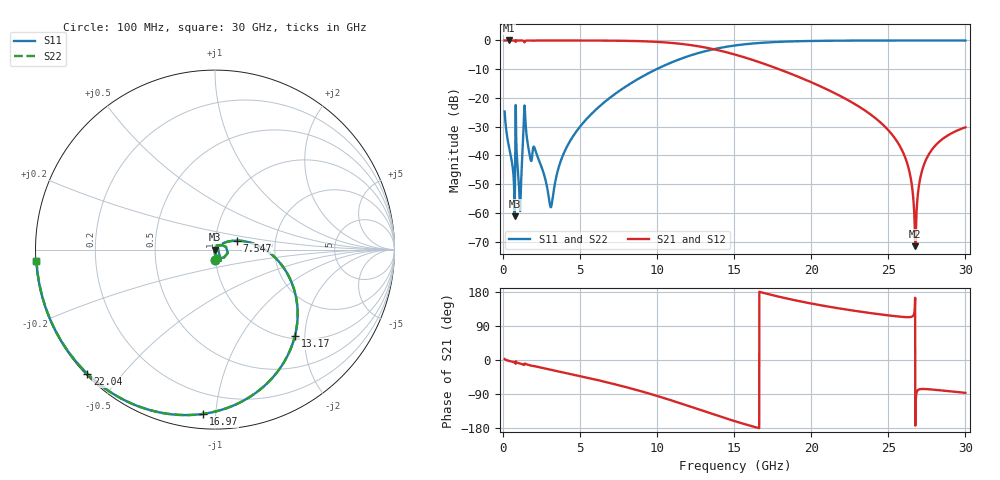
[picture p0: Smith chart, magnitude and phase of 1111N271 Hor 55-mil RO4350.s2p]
# GHz S MA R 50
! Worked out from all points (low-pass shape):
!   3201 points, 100 MHz to 30 GHz, reference 50 ohm
!   highest |S21| = 0.00 dB at 408.3 MHz (marker M1); lowest = -71.5 dB at 26.75 GHz (marker M2)
!   |S21| within 3 dB of the highest: start of sweep to 13.63 GHz
!   lowest |S11| = -61.2 dB at 754.1 MHz (marker M3), VSWR 1.00, Z = 50.1 + j0.00871 ohm
!   |S11| at or under -10 dB: start of sweep to 9.954 GHz
!   |S22| runs from -61.2 to 0.0 dB; largest |S21 - S12| = 0
!   S11 on the Smith chart (normalised r, x): 100 MHz: 1.00, -0.12; 7.547 GHz: 1.27, +0.13; 13.17 GHz: 1.06, -1.78; 16.97 GHz: 0.08, -0.93; 22.04 GHz: 0.00, -0.41; 30 GHz: 0.00, -0.03
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0.1  0.05823 -87.3  0.9981 2.5  0.9981 2.5  0.05823 -87.3
0.4083438  0.01304 -91.0  0.9995 -2.7  0.9995 -2.7  0.01304 -91.0
0.7540625  0.000874 5.7  0.9991 -6.3  0.9991 -6.3  0.000874 5.7
1.109125  0.00108 -8.7  0.9988 -9.3  0.9988 -9.3  0.00108 -8.7
1.454844  0.03839 -74.7  0.9827 -10.1  0.9827 -10.1  0.03839 -74.7
1.735156  0.009948 -86.5  0.9968 -13.9  0.9968 -13.9  0.009948 -86.5
2.11825  0.0118 -88.0  0.9959 -17.0  0.9959 -17.0  0.0118 -88.0
3.108687  0.001264 -20.0  0.9984 -25.7  0.9984 -25.7  0.001264 -20.0
3.846844  0.009507 50.4  0.9983 -32.1  0.9983 -32.1  0.009507 50.4
5.089563  0.03414 44.5  0.9975 -43.2  0.9975 -43.2  0.03414 44.5
7.546969  0.1329 22.1  0.9884 -67.1  0.9884 -67.1  0.1329 22.1
10.06978  0.3272 -6.2  0.9411 -95.7  0.9411 -95.7  0.3272 -6.2
13.17191  0.6558 -47.3  0.7493 -136.9  0.7493 -136.9  0.6558 -47.3
15.05  0.818 -71.9  0.5683 -161.6  0.5683 -161.6  0.818 -71.9
16.97481  0.9172 -94.0  0.3895 176.3  0.3895 176.3  0.9172 -94.0
20.03956  0.9797 -121.6  0.1856 148.7  0.1856 148.7  0.9797 -121.6
22.03912  0.992 -135.7  0.1029 134.7  0.1029 134.7  0.992 -135.7
25.01978  0.997 -153.2  0.02715 117.6  0.02715 117.6  0.997 -153.2
26.20644  0.9974 -159.3  0.007557 113.0  0.007557 113.0  0.9974 -159.3
26.74837  0.9974 -161.9  0.0002653 -173.4  0.0002653 -173.4  0.9974 -161.9
27.608  0.9973 -166.0  0.01027 -77.1  0.01027 -77.1  0.9973 -166.0
30  0.9968 -176.5  0.0309 -86.7  0.0309 -86.7  0.9968 -176.5
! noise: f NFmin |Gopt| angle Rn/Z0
0.1  0.0006561  0.731  1.002  0.0004861
3.417  0.009199  0.4597  28.07  0.002716
6.743  0.01514  0.4075  51.35  0.003502
10.06  0.02326  0.4503  69.75  0.005088
13.39  0.03637  0.5543  86.66  0.008291
16.7  0.06215  0.6991  105.3  0.01566
20.03  0.1256  0.8391  125.5  0.03567
23.35  0.3497  0.939  144.6  0.1196
26.67  14.09  0.9972  161.5  117
30  0.7638  0.9694  176.4  0.006982
